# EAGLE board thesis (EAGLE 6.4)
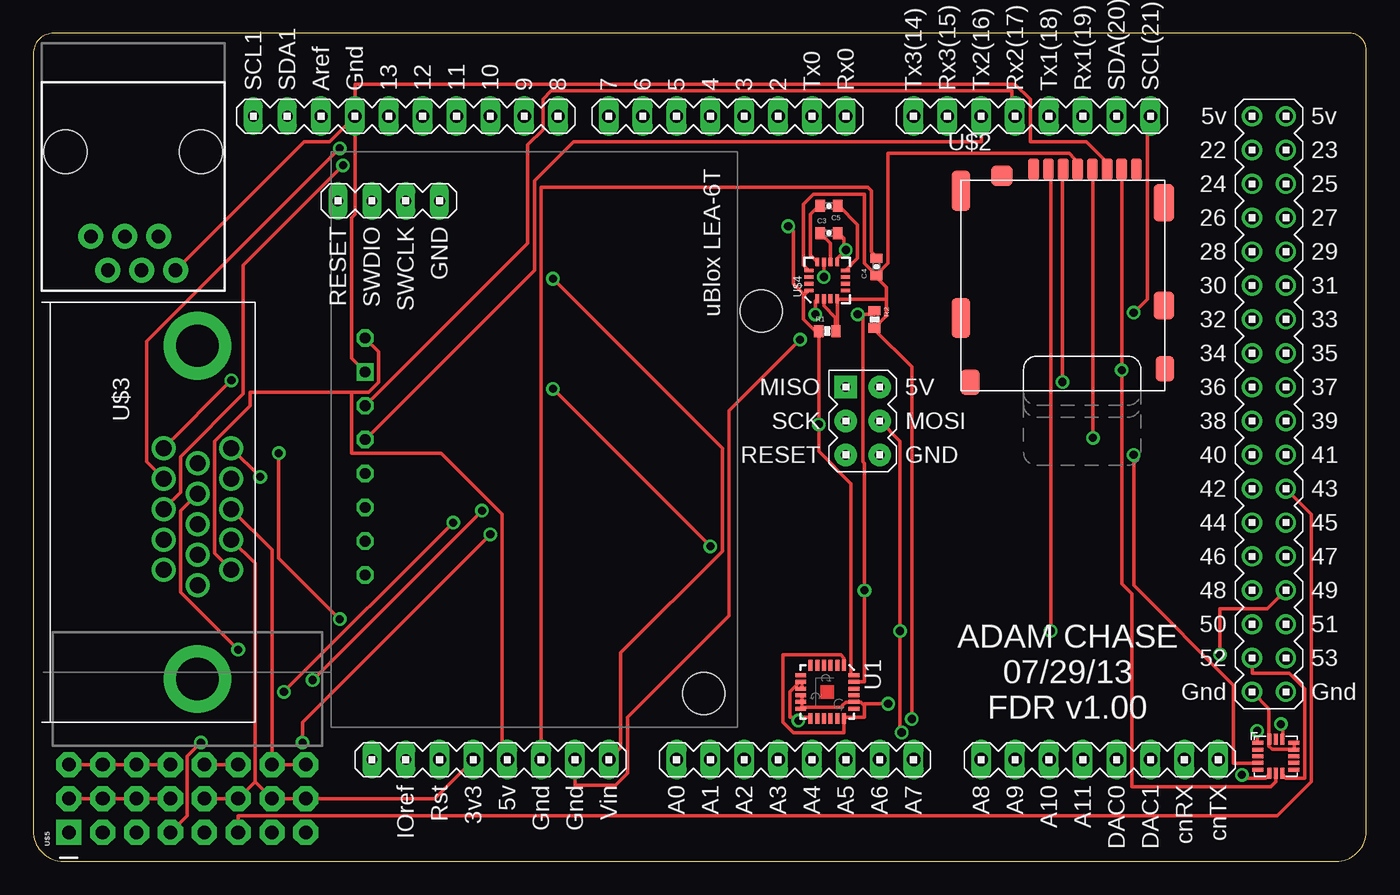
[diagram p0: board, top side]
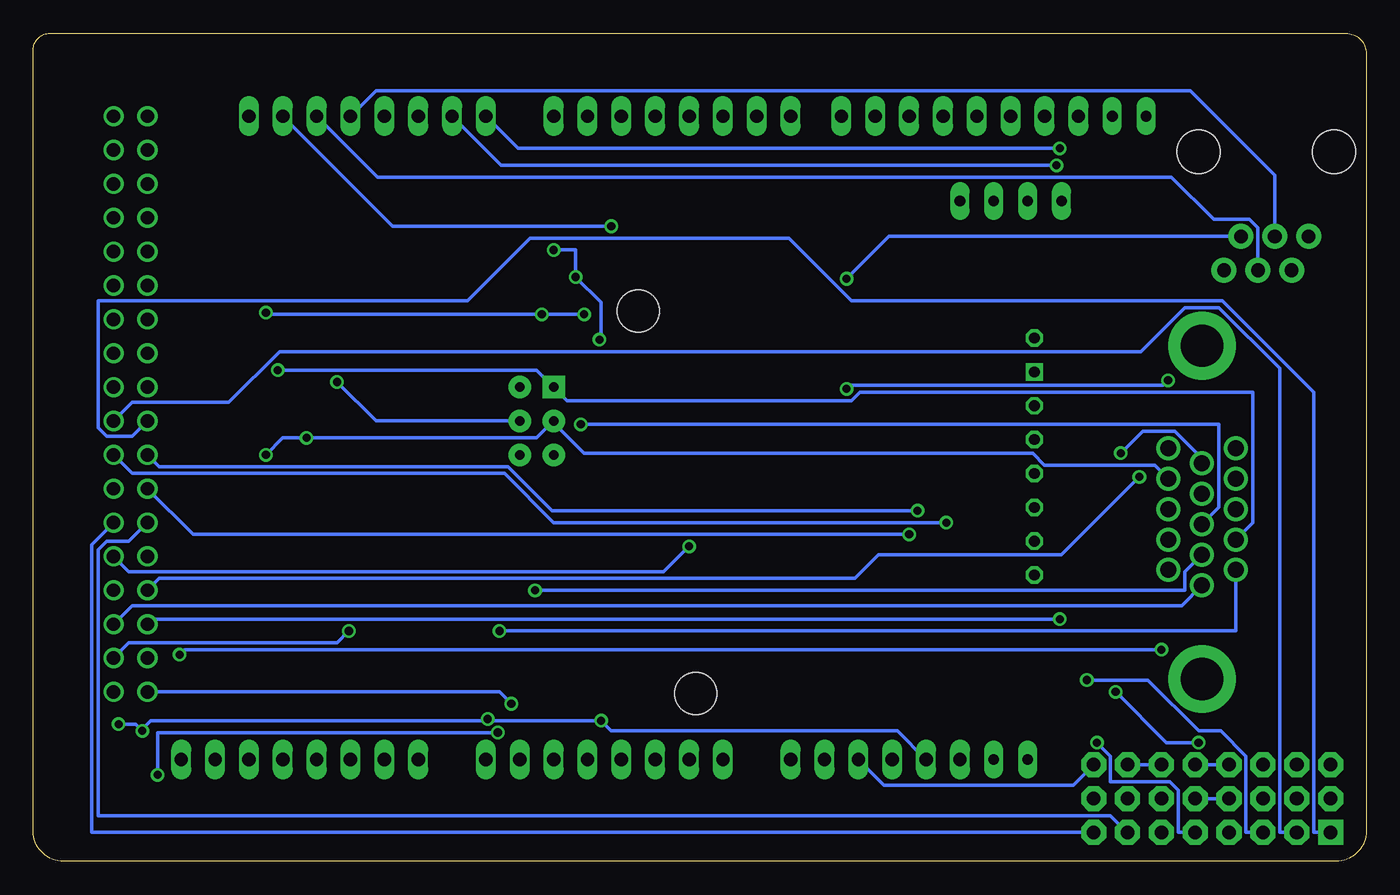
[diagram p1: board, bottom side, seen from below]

Size 100 x 62.09 mm. Coordinates in mm from the lower left corner, seen from the top.
Outline: 100,2.25 100,60.87 arc90 98.78,62.09 1.52,62.09 arc90 0,60.57 0,2.26 arc90 2.26,0 97.75,0 arc90 100,2.25
Copper layers (1*16): Top 0.035mm / dielectric 1.5mm / Bottom 0.035mm
Design rules "default": minimum track width 10mil, minimum drill 24mil, track to track 8mil, track to pad 8mil, pad to pad 8mil, via to via 8mil, smd to smd 8mil, copper to edge 40mil, drill to drill 8mil, minimum pad ring 10mil, minimum via ring 8mil, stop-mask expansion 4mil, vias tented up to drill 0mil, thermal gap 10mil
Holes 3.17 mm at 54.61,41.27

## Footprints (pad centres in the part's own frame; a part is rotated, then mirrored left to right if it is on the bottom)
SPARKFUN_0402-CAP = smd 0.7 x 0.9: 1 -0.65,0; 2 0.65,0
RJ11-6 = drill 1.016 pad 1.88: 1 1.905,8.89; 2 3.175,6.35; 3 4.445,8.89; 4 5.715,6.35; 5 6.985,8.89; 6 8.255,6.35 | hole 3.251: 0,0; 10.16,0
SPARKFUN_0402-RES = smd 0.7 x 0.9: 1 -0.65,0; 2 0.65,0
QFN-24 = smd 0.8 x 0.3: 1 -2,1.25; 2 -2,0.75; 3 -2,0.25; 4 -2,-0.25; 5 -2,-0.75; 6 -2,-1.25; 13 2,-1.25; 14 2,-0.75; 15 2,-0.25; 16 2,0.25; 17 2,0.75; 18 2,1.25 | smd 0.3 x 0.8: 7 -1.25,-2; 8 -0.75,-2; 9 -0.25,-2; 10 0.25,-2; 11 0.75,-2; 12 1.25,-2; 19 1.25,2; 20 0.75,2; 21 0.25,2; 22 -0.25,2; 23 -0.75,2; 24 -1.25,2
ADXL362 = smd 0.8 x 0.3: P$1 -1.35,1; P$2 -1.35,0.5; P$3 -1.35,0; P$4 -1.35,-0.5; P$5 -1.35,-1; P$9 1.35,-1; P$10 1.35,-0.5; P$11 1.35,0; P$12 1.35,0.5; P$13 1.35,1 | smd 0.3 x 0.8: P$6 -0.5,-1.275; P$7 0,-1.275; P$8 0.5,-1.275; P$14 0.5,1.275; P$15 0,1.275; P$16 -0.5,1.275
DUE(NORMAL) = drill 1 long: 2 -16.51,30.48; 3 -19.05,30.48; 3V3 -39.37,-17.78; 4 -21.59,30.48; 5 -24.13,30.48; 5V -36.83,-17.78; 6 -26.67,30.48; 7 -29.21,30.48; 8 -33.02,30.48; 9 -35.56,30.48; 10 -38.1,30.48; 11 -40.64,30.48; 12 -43.18,30.48; 13 -45.72,30.48; A0 -24.13,-17.78; A1 -21.59,-17.78; A2 -19.05,-17.78; A3 -16.51,-17.78; A4 -13.97,-17.78; A5 -11.43,-17.78; A6 -8.89,-17.78; A7 -6.35,-17.78; A8 -1.27,-17.78; A9 1.27,-17.78; A10 3.81,-17.78; A11 6.35,-17.78; AREF -50.8,30.48; AREF1 -50.8,30.48; CANRX 13.97,-17.78; CANTX 16.51,-17.78; DAC0 8.89,-17.78; DAC1 11.43,-17.78; GND1 -48.26,30.48; GND_1 -34.29,-17.78; GND_2 -31.75,-17.78; RESET -41.91,-17.78; RX0 -11.43,30.48; RX1 6.35,30.48; RX2 1.27,30.48; RX3 -3.81,30.48; SCL 11.43,30.48; SDA 8.89,30.48; TX0 -13.97,30.48; TX1 3.81,30.48; TX2 -1.27,30.48; TX3 -6.35,30.48; VIN -29.21,-17.78 | drill 1: 5V_A 19.05,30.48; 5V_B 21.59,30.48; 22 19.05,27.94; 23 21.59,27.94; 24 19.05,25.4; 25 21.59,25.4; 26 19.05,22.86; 27 21.59,22.86; 28 19.05,20.32; 29 21.59,20.32; 30 19.05,17.78; 31 21.59,17.78; 32 19.05,15.24; 33 21.59,15.24; 34 19.05,12.7; 35 21.59,12.7; 36 19.05,10.16; 37 21.59,10.16; 38 19.05,7.62; 39 21.59,7.62; 40 19.05,5.08; 41 21.59,5.08; 42 19.05,2.54; 43 21.59,2.54; 44 19.05,0; 45 21.59,0; 46 19.05,-2.54; 47 21.59,-2.54; 48 19.05,-5.08; 49 21.59,-5.08; 50 19.05,-7.62; 51 21.59,-7.62; 52 19.05,-10.16; 53 21.59,-10.16; GND_A 19.05,-12.7; GND_B 21.59,-12.7 | drill 0.7 pad 1.676: 5V_ICSP -8.89,5.08; GND_ICSP -8.89,10.16; MOSI_ICSP -8.89,7.62; RESET_ICSP -11.43,5.08; SCK_ICSP -11.43,7.62 | drill 0.8 pad 1.422 long: GND_DEBUG -41.91,24.13; IOREF -44.45,-17.78; NC -46.99,-17.78; RESET_DEBUG -49.53,24.13; SCL1 -55.88,30.48; SDA1 -53.34,30.48; SWCLK_DEBUG -44.45,24.13; SWDIO_DEBUG -46.99,24.13 | drill 0.7 pad 1.676 square: MISO_ICSP -11.43,10.16
MICRO_SD_CONNECTOR = smd 0.8 x 1.6: 1 -2.03,8.2; 2 -0.93,8.2; 3 0.17,8.2; 4 1.27,8.2; 5 2.37,8.2; 6 3.47,8.2; 7 4.57,8.2; 8 5.67,8.2 | smd 1.55 x 2.8: 9 7.735,5.7 | smd 1.55 x 2.1: 10 7.735,-2 | smd 1.4 x 1.9: 11 7.81,-6.75; 12 -6.79,-7.75 | smd 1.4 x 3: 13 -7.49,-2.95; 14 -7.49,6.6 | smd 1.6 x 1.55: 15 -4.43,7.725
DB-15-F90+SHIELD-SMALL_PADS = drill 1.2 pad 1.524: 1 4.318,14.224; 2 2.032,14.224; 3 -0.254,14.224; 4 -2.54,14.224; 5 -4.826,14.224; 6 5.461,11.684; 7 3.175,11.684; 8 0.889,11.684; 9 -1.397,11.684; 10 -3.683,11.684; 11 4.318,9.144; 12 2.032,9.144; 13 -0.254,9.144; 14 -2.54,9.144; 15 -4.826,9.144 | drill 3.175 pad 5.08: SHIELD@1 -12.497,11.684; SHIELD@2 12.497,11.684
SPARKFUN_16LPCC = smd 0.65 x 0.28: 1 -1.37,0.75; 2 -1.37,0.25; 3 -1.37,-0.25; 4 -1.37,-0.75; 9 1.37,-0.75; 10 1.37,-0.25; 11 1.37,0.25; 12 1.37,0.75 | smd 0.28 x 0.65: 5 -0.75,-1.37; 6 -0.25,-1.37; 7 0.25,-1.37; 8 0.75,-1.37; 13 0.75,1.37; 14 0.25,1.37; 15 -0.25,1.37; 16 -0.75,1.37
3X8RA = drill 1.016 pad 1.88 square: 1 -1.27,8.89 | drill 1.016 pad 1.88 octagon: 2 1.27,8.89; 3 3.81,8.89; 4 -1.27,6.35; 5 1.27,6.35; 6 3.81,6.35; 7 -1.27,3.81; 8 1.27,3.81; 9 3.81,3.81; 10 -1.27,1.27; 11 1.27,1.27; 12 3.81,1.27; 13 -1.27,-1.27; 14 1.27,-1.27; 15 3.81,-1.27; 16 -1.27,-3.81; 17 1.27,-3.81; 18 3.81,-3.81; 19 -1.27,-6.35; 20 1.27,-6.35; 21 3.81,-6.35; 22 -1.27,-8.89; 23 1.27,-8.89; 24 3.81,-8.89
UBLOXLEA6TBOB = drill 0.8 octagon: 5V 13.97,2.54; RS232DI 24.13,2.54; RS232DO 26.67,2.54; TIMEOUT1 29.21,2.54; TIMEOUT2 31.75,2.54; TTLDI 21.59,2.54; TTLDO 19.05,2.54 | drill 0.8 square: GND 16.51,2.54 | hole 3.175: 40.64,27.94

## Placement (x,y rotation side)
C3  4.7uF  [SPARKFUN_0402-CAP]  59.69,47.12 0 top
C4  0.1uF  [SPARKFUN_0402-CAP]  63.25,44.58 90 top
C5  0.22uF  [SPARKFUN_0402-CAP]  59.69,49.15 180 top
J1  RJ11-6PTH  [RJ11-6]  12.57,53.21 180 top
R1  4.7K  [SPARKFUN_0402-RES]  59.56,39.75 0 top
R2  4.7K  [SPARKFUN_0402-RES]  63.12,40.64 270 top
U1  ITG-3200  [QFN-24]  59.56,12.7 270 top
U2  ADXL362  [ADXL362]  93.22,7.87 0 top
U$1  DUE(NORMAL)  [DUE(NORMAL)]  72.39,25.4 0 top
U$2  MICROSD_SPI_MODE  [MICRO_SD_CONNECTOR]  77.09,43.69 0 top
U$3  VGA-F90S  [DB-15-F90+SHIELD-SMALL_PADS]  0.64,26.16 270 top
U$4  SPARKFUN_HMC5883LSMD  [SPARKFUN_16LPCC]  59.56,43.56 90 top
U$5  HEADER-3X8SERVO  [3X8RA]  11.56,3.43 90 top
U$6  UBLOXLEA6TBOB  [UBLOXLEA6TBOB]  22.35,53.21 270 top

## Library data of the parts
C3-C5 R1 R2 U$4 = HMC5883L_Breakout-v11
J1 = SparkFun-Connectors
U1 = SparkFun
U2 = SparkFun-Sensors; PROD_ID: IC-11297
U$1 = DUElib130425
U$2 = con-molex-microsd
U$3 = VideoConnectors
U$5 = pixhawk2
U$6 = csgshop

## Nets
5V: U$1.5V U$3.1 U$6.5V
33V: C4.1 R1.2 R2.2 U1.8 U1.9 U1.13 U2.P$1 U2.P$14 U$1.3V3 U$2.4 U$3.2 U$4.2 U$4.4 U$4.13 U$5.2 U$5.5 U$5.8 U$5.11 U$5.14 U$5.17 U$5.20 U$5.23
D47: U$1.47 U$3.15
D48: U$1.48 U$3.5
D49: U$1.49 U$3.9
D50: U$1.50 U$3.10
D51: U$1.51 U$3.6
D52: U2.P$8 U$1.52
D53: U$1.53 U$2.2
GND1: C4.2 U$1.GND_1 U$3.3 U$5.3 U$5.6 U$5.9 U$5.12 U$5.15 U$5.18 U$5.21 U$5.24
GND1_1: J1.1 U$1.GND1 U$2.6 U$6.GND
GND2: C3.2 U$1.GND_2 U$4.9 U$4.11
GNDA: U1.1 U1.10 U1.11 U1.12 U1.18 U1.20 U2.P$12 U2.P$13 U2.P$16 U$1.GND_A
MISO: U2.P$7 U$1.MISO_ICSP U$2.7 U$3.12
MOSI: U2.P$6 U$1.MOSI_ICSP U$2.3 U$3.11
N$1: U$1.38 U$5.1
N$2: U$1.39 U$5.4
N$3: U$1.40 U$5.7
N$4: U$1.41 U$5.10
N$5: C5.1 U$4.8
N$6: U$1.42 U$5.13
N$7: C5.2 U$4.12
N$8: U$1.43 U$5.16
N$9: U$1.44 U$5.19
N$10: U$1.45 U$5.22
N$12: C3.1 U$4.10
RX1: J1.3 U$1.RX1
RX2: U$1.RX2 U$6.TTLDO
RX3: U$1.RX3 U$3.13
SCL: R2.1 U1.23 U$1.SCL U$3.7 U$4.1
SCLK: U2.P$4 U$1.SCK_ICSP U$2.5 U$3.4
SDA: R1.1 U1.24 U$1.SDA U$3.8 U$4.16
TX1: J1.4 U$1.TX1
TX2: U$1.TX2 U$6.TTLDI
TX3: U$1.TX3 U$3.14
VIN: J1.2 U$1.VIN

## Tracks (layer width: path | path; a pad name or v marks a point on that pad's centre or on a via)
5V
  Top 0.254: U$6.5V 25.91,38.23 25.91,35.94 25.15,35.18 23.88,35.18 | 23.88,35.18 16.26,35.18 16.26,34.16 13.59,31.5 13.59,23.11 U$3.1 | U$1.5V 35.18,8 35.18,26.04 30.61,30.61 23.88,30.61 23.88,35.18
33V  (via drill 0.61)
  Top 0.254: U$1.3V3 30.1,4.7 U$5.23 U$5.20 16.64,5.97 | U$5.2 U$5.5 U$5.8 U$5.11 | U$3.2 16.64,22.35 16.64,5.97 | 16.64,5.97 U$5.17 U$5.14 | U$4.2 59.31,42.16 59.31,41.66 60.2,40.77 60.2,39.75 R1.2 60.33,39.75 60.33,42.16 U$4.4 60.45,42.16 64.01,42.16 | 63.25,43.94 62.36,44.83 62.36,50.04 58.55,50.04 57.78,49.28 57.78,44.7 58.17,44.32 U$4.13 | 64.01,42.16 64.01,43.05 63.25,43.81 C4.1 63.25,43.94 | 64.01,42.16 64.01,40.89 63.12,40.01 R2.2 63.12,39.88 65.91,37.08 v65.91,10.67 | 63.25,43.94 64.14,44.83 64.14,53.09 77.72,53.09 78.11,52.7 78.11,52.2 78.36,51.94 U$2.4 | v91.82,9.78 91.82,8.89 U2.P$1 | v93.6,10.29 93.73,10.16 93.73,9.27 U2.P$14 | U1.9 57.66,12.95 57.66,13.34 U1.8 57.53,13.46 56.77,12.7 56.77,10.79 57.4,10.79 | 57.4,10.79 58.29,10.79 U1.13 | 57.4,10.79 v57.4,10.54
  Bottom 0.254: U$5.14 U$5.11 | v93.6,10.29 92.33,10.29 v91.82,9.78 91.82,9.91 91.19,10.54 65.91,10.54 | 65.91,10.54 v57.4,10.54 56.64,9.78 35.18,9.78 U$1.3V3 | 65.91,10.54 v65.91,10.67
D47  (via drill 0.61)
  Top 0.254: v38.99,35.43 v50.8,23.62 | U$3.15 v14.86,36.07
  Bottom 0.254: U$1.47 92.84,21.72 52.7,21.72 v50.8,23.62 | v38.99,35.43 38.73,35.69 15.24,35.69 v14.86,36.07
D48  (via drill 0.61)
  Top 0.254: U$3.5 v17.02,28.83
  Bottom 0.254: U$1.48 90.55,21.21 38.35,21.21 36.58,22.99 22.86,22.99 v17.02,28.83
D49  (via drill 0.61)
  Top 0.254: U$1.49 92.58,18.92 89.03,18.92 v89.03,15.49 | v15.37,15.88 11.05,20.19 11.05,26.29 U$3.9
  Bottom 0.254: v89.03,15.49 88.65,15.88 v15.37,15.88
D50  (via drill 0.61)
  Top 0.254: v22.99,18.16 18.41,22.73 v18.41,30.61
  Bottom 0.254: U$1.50 91.06,18.16 v22.99,18.16 | v18.41,30.61 16.76,32.26 14.35,32.26 12.32,30.23 U$3.10
D51
  Bottom 0.254: U$1.51 92.58,19.18 13.84,19.18 U$3.6
D52
  Top 0.254: U$1.52 91.44,14.1 94.23,14.1 95.38,12.95 95.38,6.22 93.98,6.22 93.73,6.48 U2.P$8
D53  (via drill 0.61)
  Top 0.254: v76.33,17.27 76.33,51.69 76.2,51.82 U$2.2
  Bottom 0.254: v76.33,17.27 77.22,16.38 92.84,16.38 U$1.53
GND1
  Top 0.254: U$5.18 U$5.15 | U$5.3 U$5.6 U$5.9 U$5.12 | U$3.3 17.91,23.37 U$5.21 U$5.24 | U$1.GND_1 38.1,50.55 62.61,50.55 62.87,50.29 62.87,45.72 63.25,45.34 C4.2
  Bottom 0.254: U$5.12 U$5.15 | U$5.21 U$5.18 | U$5.24 21.97,5.71 36.2,5.71 U$1.GND_1
GND1_1
  Top 0.254: U$1.GND1 24.13,58.29 73.66,58.29 74.8,57.15 74.8,53.98 78.99,53.98 80.26,52.7 80.26,52.2 80.52,51.94 U$2.6 | U$6.GND 23.88,37.72 23.88,48.26 24.13,48.51 U$1.GND1 | J1.1 20.32,53.98 22.23,53.98 U$1.GND1
GND2  (via drill 0.61)
  Top 0.254: v59.31,43.81 59.31,44.83 U$4.11 | U$4.9 60.33,44.96 60.33,45.21 v60.96,45.85 60.83,45.85 60.83,46.74 60.45,47.12 C3.2 | v57.53,39.12 52.2,33.78 52.2,18.41 44.58,10.79 44.58,6.6 43.69,5.71 40.64,5.71 U$1.GND_2
  Bottom 0.254: v60.96,45.85 59.31,45.85 v59.31,43.81 57.4,41.91 57.4,39.12 v57.53,39.12
GNDA  (via drill 0.61)
  Top 0.254: U1.10 57.66,12.45 57.66,12.06 U1.11 57.66,11.94 57.66,11.56 U1.12 57.78,11.56 60.71,11.56 60.71,11.68 60.96,11.94 61.47,11.94 U1.20 61.59,11.94 62.1,11.94 62.29,11.75 | 62.29,11.75 62.36,11.68 62.36,10.79 60.83,10.79 U1.18 60.83,10.67 60.83,9.65 57.02,9.65 56.26,10.41 56.26,15.49 60.58,15.49 60.83,15.24 60.83,14.73 U1.1 | U2.P$13 94.61,8.76 94.61,8.38 U2.P$12 94.49,8.38 92.96,8.38 92.71,8.64 U2.P$16 92.71,9.27 92.71,11.43 U$1.GND_A | v64.14,11.81 62.36,11.81 62.29,11.75
  Bottom 0.254: v64.14,11.81 65.02,12.7 U$1.GND_A
MISO  (via drill 0.61)
  Top 0.254: U2.P$7 93.22,5.97 92.84,5.59 82.42,5.59 82.42,20.07 81.66,20.83 v81.66,36.83 81.66,51.82 U$2.7
  Bottom 0.254: v81.66,36.83 62.23,36.83 U$1.MISO_ICSP 59.94,34.54 38.61,34.54 37.97,35.18 8.51,35.18 8.51,25.4 U$3.12
MOSI  (via drill 0.61)
  Top 0.254: v90.68,6.48 90.68,6.22 92.46,6.22 92.71,6.48 U2.P$6 | v65.15,9.65 65.02,9.78 v65.02,17.27 65.02,31.5 U$1.MOSI_ICSP | v77.22,35.94 77.22,51.82 U$2.3
  Bottom 0.254: v90.68,6.48 90.68,9.65 v65.15,9.65 | v77.22,35.94 74.3,33.02 U$1.MOSI_ICSP | U$3.11 9.78,17.27 v65.02,17.27
N$1
  Bottom 0.254: U$1.38 92.58,31.88 94.49,31.88 95.12,32.51 95.12,42.04 67.44,42.04 62.74,46.74 43.31,46.74 38.61,42.04 10.79,42.04 3.94,35.18 3.94,2.16 U$5.1
N$2
  Bottom 0.254: U$1.39 92.58,34.42 85.34,34.42 81.53,38.23 16.89,38.23 13.59,41.53 11.05,41.53 6.48,36.96 6.48,2.16 U$5.4
N$3  (via drill 0.61)
  Top 0.254: v20.95,13.59 v33.66,26.29
  Bottom 0.254: U$1.40 90.55,29.59 64.39,29.59 61.09,26.29 v33.66,26.29 | v20.95,13.59 16.38,13.59 12.57,9.78 10.92,9.78 9.02,7.87 9.02,2.16 U$5.7
N$4  (via drill 0.61)
  Top 0.254: v18.8,12.7 v31.5,25.4 | v12.57,8.89 11.56,7.87 11.56,3.43 U$5.10
  Bottom 0.254: U$1.41 92.58,29.08 64.64,29.08 60.96,25.4 v31.5,25.4 | v18.8,12.7 14.99,8.89 v12.57,8.89
N$5
  Top 0.254: U$4.8 60.96,44.32 61.85,45.21 61.85,47.75 60.45,49.15 C5.1
N$6  (via drill 0.61)
  Top 0.254: v34.29,24.51 20.19,10.41 v20.19,8.89
  Bottom 0.254: U$1.42 88.01,24.51 v34.29,24.51 | v20.19,8.89 19.18,7.87 19.18,5.97 14.73,5.97 14.1,5.33 14.1,2.16 U$5.13
N$7
  Top 0.254: U$4.12 58.8,44.96 58.29,45.47 58.29,48.51 58.93,49.15 C5.2
N$8
  Top 0.254: U$1.43 95.89,26.04 95.89,5.97 93.34,3.43 15.37,3.43 U$5.16
N$9
  Bottom 0.254: U$1.44 92.84,24 94.49,24 95.12,23.37 95.12,3.43 19.18,3.43 U$5.19
N$10
  Bottom 0.254: U$1.45 95.63,23.75 95.63,2.16 U$5.22
N$12
  Top 0.254: U$4.10 59.82,44.96 59.82,46.35 59.05,47.12 C3.1
RX1
  Bottom 0.254: U$1.RX1 74.17,51.31 14.61,51.31 11.43,48.13 8.76,48.13 8.13,47.5 J1.3
RX2
  Top 0.254: U$6.TTLDO 37.08,46.35 37.08,53.72 38.23,54.86 38.23,57.15 38.86,57.78 73.41,57.78 73.41,56.13 U$1.RX2
RX3  (via drill 0.61)
  Top 0.254: v23.24,52.2 15.75,44.7 15.75,35.05 11.05,30.35 11.05,27.69 U$3.13
  Bottom 0.254: U$1.RX3 64.9,52.2 v23.24,52.2
SCL  (via drill 0.61)
  Top 0.254: v58.67,41.02 58.67,42.04 58.8,42.16 U$4.1 | 62.23,41.02 63.12,41.02 R2.1 | 62.23,41.02 62.23,29.97 62.36,29.84 v62.36,20.32 62.36,13.46 61.59,13.46 U1.23 | 62.23,41.02 v61.85,41.02 | U$1.SCL 83.57,55.63 83.57,42.16 v82.55,41.15
  Bottom 0.254: v58.67,41.02 v61.85,41.02 82.42,41.02 v82.55,41.15 | U$3.7 13.59,21.72 13.59,20.32 v62.36,20.32
SCLK  (via drill 0.61)
  Top 0.254: v82.55,30.48 82.55,20.7 90.04,13.21 90.04,7.37 91.82,7.37 U2.P$4 | v79.5,31.75 79.5,51.82 U$2.5
  Bottom 0.254: v82.55,30.48 81.28,31.75 v79.5,31.75 62.23,31.75 U$1.SCK_ICSP 60.96,32.89 58.67,30.61 25.02,30.61 24.13,29.72 15.88,29.72 U$3.4
SDA  (via drill 0.61)
  Top 0.254: 57.85,42.48 57.78,42.42 57.78,40.64 58.67,39.75 R1.1 58.93,39.75 v58.93,32.77 58.93,30.73 61.34,28.32 61.34,14.1 61.47,13.97 U1.24 | 57.85,42.48 58.17,42.8 U$4.16 | v56.64,47.62 57.02,47.24 57.02,43.31 57.85,42.48
  Bottom 0.254: U$1.SDA 73.03,47.62 v56.64,47.62 | U$3.8 11.05,26.54 11.05,32.77 v58.93,32.77
TX1
  Bottom 0.254: U$1.TX1 74.3,57.78 13.21,57.78 6.86,51.44 J1.4
TX2
  Top 0.254: U$6.TTLDI 37.59,44.32 37.59,51.05 40.51,53.98 71.12,53.98 U$1.TX2
TX3  (via drill 0.61)
  Top 0.254: v22.99,53.47 8.51,38.99 8.51,29.97 U$3.14
  Bottom 0.254: U$1.TX3 63.63,53.47 v22.99,53.47
VIN  (via drill 0.61)
  Top 0.254: U$1.VIN 44.07,8.51 44.07,15.62 51.69,23.24 51.69,30.99 v38.99,43.69
  Bottom 0.254: v38.99,43.69 35.81,46.86 J1.2

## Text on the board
tPlace: ADAM CHASE / 07/29/13 / FDR v1.00

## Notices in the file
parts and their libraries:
SparkFun-Sensors: Licensing: CC v3.0 Share-Alike You are welcome to use this library for commercial purposes.
